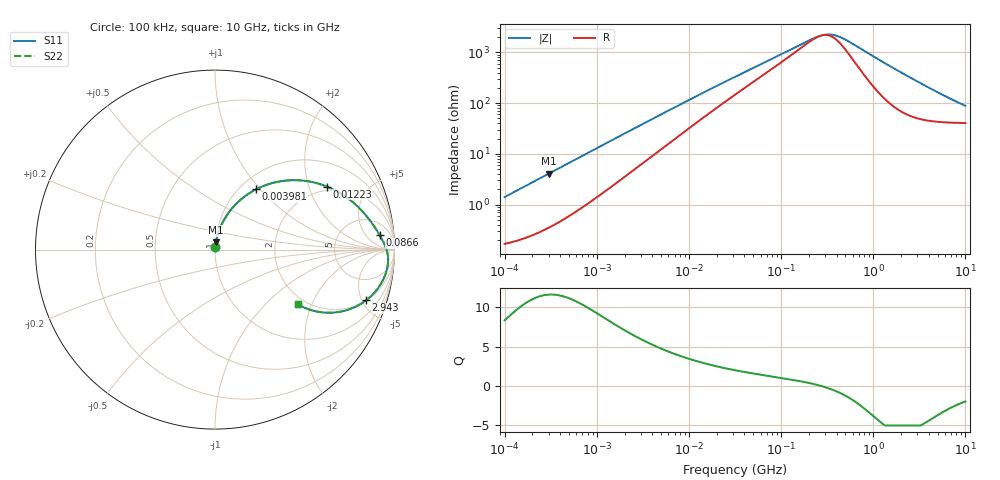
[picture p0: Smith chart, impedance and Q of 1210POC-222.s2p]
# MHz S MA R 50
!Freq  MagS11  AngS11  MagS21  AngS21  MagS12  AngS12  MagS22  AngS22
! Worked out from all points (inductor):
!   801 points, 100 kHz to 10 GHz, reference 50 ohm
!   read as one part in series: L = 2.21 uH near 105.9 kHz
!   highest Q = 11.6 at 302.9 kHz (marker M1), where L = 2.15 uH
!   self-resonance near 275 MHz
!   S11 on the Smith chart (normalised r, x): 100 kHz: 1.00, +0.03; 3.981 MHz: 1.18, +0.95; 12.23 MHz: 1.84, +2.65; 86.6 MHz: 12, +12; 2.943 GHz: 2.02, -5.39; 10 GHz: 1.81, -1.58
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0.1  0.01407 82.4  0.9982 -0.8  0.9982 -0.8  0.01407 82.4
0.3028656  0.0408 82.8  0.9957 -2.3  0.9957 -2.3  0.0408 82.8
0.6878599  0.08921 79.4  0.9875 -5.1  0.9875 -5.1  0.08921 79.4
1.883649  0.2245 69.3  0.9444 -12.8  0.9444 -12.8  0.2245 69.3
2.778114  0.3108 62.9  0.902 -17.9  0.902 -17.9  0.3108 62.9
3.981072  0.4076 55.6  0.8402 -23.6  0.8402 -23.6  0.4076 55.6
4.663908  0.4538 52.1  0.805 -26.4  0.805 -26.4  0.4538 52.1
7.498942  0.5932 40.7  0.6726 -35.1  0.6726 -35.1  0.5932 40.7
12.23207  0.7159 29.4  0.5147 -43.0  0.5147 -43.0  0.7159 29.4
19.38653  0.799 20.5  0.3764 -48.0  0.3764 -48.0  0.799 20.5
31.62278  0.857 13.5  0.2597 -50.1  0.2597 -50.1  0.857 13.5
86.59643  0.9212 5.0  0.1144 -44.1  0.1144 -44.1  0.9212 5.0
217.5204  0.9508 0.9  0.0514 -16.3  0.0514 -16.3  0.9508 0.9
307.2557  0.958 -0.4  0.04259 9.4  0.04259 9.4  0.958 -0.4
354.8134  0.9605 -1.0  0.04283 22.2  0.04283 22.2  0.9605 -1.0
409.7321  0.9626 -1.5  0.04575 34.4  0.04575 34.4  0.9626 -1.5
530.8844  0.9655 -2.7  0.05737 51.6  0.05737 51.6  0.9655 -2.7
1474.857  0.9537 -9.7  0.1721 69.6  0.1721 69.6  0.9537 -9.7
2113.489  0.9296 -13.9  0.2431 66.4  0.2431 66.4  0.9296 -13.9
2942.727  0.888 -18.5  0.3237 60.8  0.3237 60.8  0.888 -18.5
5463.865  0.743 -28.2  0.4925 45.5  0.4925 45.5  0.743 -28.2
10000  0.5513 -33.5  0.62 29.4  0.62 29.4  0.5513 -33.5
